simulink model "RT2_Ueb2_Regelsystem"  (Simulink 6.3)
settings: Solver=ode45  StartTime=0.0  StopTime=tfin  RelTol=1e-3
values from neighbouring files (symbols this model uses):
  a = ###    [RT2_Ueb2A1.m]
  b = 1    [RT2_Ueb2A1.m]
  c = 0    [RT2_Ueb2A1.m]
  kp = ###    [RT2_Ueb2A1.m]    (also in RT2_Ueb2A2.m)
  Td = ###    [RT2_Ueb2A1.m]    (also in RT2_Ueb2A2.m = 1/2*(tan(psi-phip)*(rps/rp-phips*tan(phi-phip))+     tan(phi)
  Ti = ###    [RT2_Ueb2A1.m]    (also in RT2_Ueb2A2.m = 1/(Td*wc^2-tan(phi-phip)*wc))
  u_low = -4    [RT2_Ueb2A1.m]
  u_up = 4    [RT2_Ueb2A1.m]
libraries: cstblocks x3

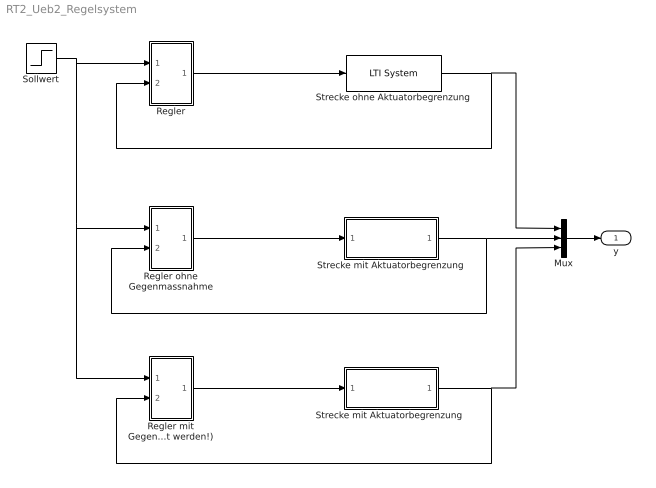
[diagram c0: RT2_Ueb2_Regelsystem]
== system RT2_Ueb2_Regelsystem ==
  Mux : Mux  Inputs=3
  Regler : Subsystem
  Regler mit Gegenmassnahme (Nur dieser Block muss verändert werden!) : Subsystem
  Regler ohne Gegenmassnahme : Subsystem
  Sollwert : Step  Time=0  SampleTime=.1
  Strecke mit Aktuatorbegrenzung : Subsystem
  "Strecke mit Aktuatorbegrenzung " : Subsystem
  Strecke ohne Aktuatorbegrenzung : cstblocks/LTI System  sys=P  IC=[]
  y : Outport
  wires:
  Strecke ohne Aktuatorbegrenzung/1 -> Regler/2(y), Mux/1
  Sollwert/1 -> Regler/1(r), Regler mit Gegenmassnahme (Nur dieser Block muss verändert werden!)/1(r), Regler ohne Gegenmassnahme/1(r)
  Regler/1(u) -> Strecke ohne Aktuatorbegrenzung/1
  "Strecke mit Aktuatorbegrenzung "/1(y) -> Regler mit Gegenmassnahme (Nur dieser Block muss verändert werden!)/2(y), Mux/3
  Regler mit Gegenmassnahme (Nur dieser Block muss verändert werden!)/1(u) -> "Strecke mit Aktuatorbegrenzung "/1(u)
  Strecke mit Aktuatorbegrenzung/1(y) -> Regler ohne Gegenmassnahme/2(y), Mux/2
  Regler ohne Gegenmassnahme/1(u) -> Strecke mit Aktuatorbegrenzung/1(u)
  Mux/1 -> y/1

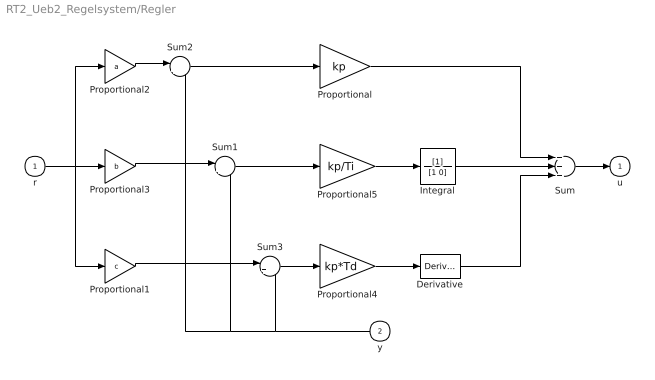
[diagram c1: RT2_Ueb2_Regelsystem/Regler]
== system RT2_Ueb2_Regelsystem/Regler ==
  r : Inport
  y : Inport  Orientation=left  Port=2
  Derivative : Derivative
  Integral : TransferFcn  Denominator=[1 0]
  Proportional : Gain  Gain=kp
  Proportional1 : Gain  Gain=c
  Proportional2 : Gain  Gain=a
  Proportional3 : Gain  Gain=b
  Proportional4 : Gain  Gain=kp*Td
  Proportional5 : Gain  Gain=kp/Ti
  Sum : Sum  Inputs=+++
  Sum1 : Sum  Inputs=|+-
  Sum2 : Sum  Inputs=|+-
  Sum3 : Sum  Inputs=|+-
  u : Outport  InitialOutput=0
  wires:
  Proportional/1 -> Sum/1
  Integral/1 -> Sum/2
  Derivative/1 -> Sum/3
  Sum1/1 -> Proportional5/1
  Sum/1 -> u/1
  Proportional4/1 -> Derivative/1
  r/1 -> Proportional2/1, Proportional1/1, Proportional3/1
  Sum2/1 -> Proportional/1
  Proportional2/1 -> Sum2/1
  Proportional1/1 -> Sum3/1
  Proportional3/1 -> Sum1/1
  Proportional5/1 -> Integral/1
  Sum3/1 -> Proportional4/1
  y/1 -> Sum3/2, Sum1/2, Sum2/2

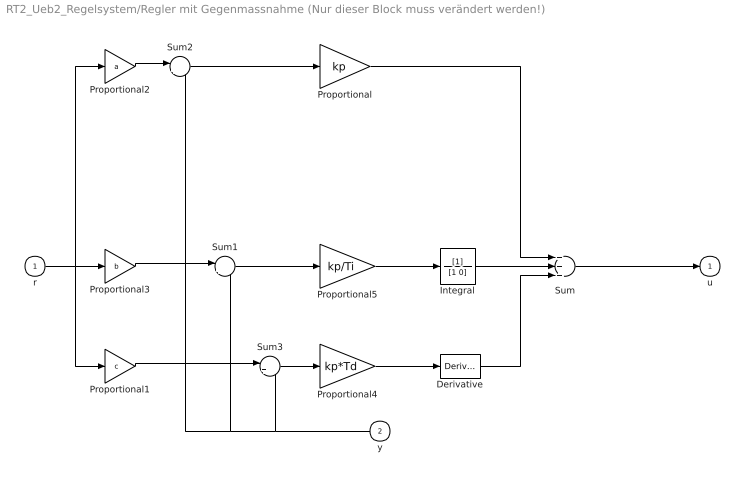
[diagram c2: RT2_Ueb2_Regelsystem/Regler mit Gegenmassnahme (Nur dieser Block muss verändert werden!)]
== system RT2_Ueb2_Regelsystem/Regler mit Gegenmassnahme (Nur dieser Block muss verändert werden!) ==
  r : Inport
  y : Inport  Orientation=left  Port=2
  Derivative : Derivative
  Integral : TransferFcn  Denominator=[1 0]
  Proportional : Gain  Gain=kp
  Proportional1 : Gain  Gain=c
  Proportional2 : Gain  Gain=a
  Proportional3 : Gain  Gain=b
  Proportional4 : Gain  Gain=kp*Td
  Proportional5 : Gain  Gain=kp/Ti
  Sum : Sum  Inputs=+++
  Sum1 : Sum  Inputs=|+-
  Sum2 : Sum  Inputs=|+-
  Sum3 : Sum  Inputs=|+-
  u : Outport  InitialOutput=0
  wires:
  y/1 -> Sum2/2, Sum1/2, Sum3/2
  Sum3/1 -> Proportional4/1
  Proportional5/1 -> Integral/1
  Proportional3/1 -> Sum1/1
  Proportional1/1 -> Sum3/1
  Proportional2/1 -> Sum2/1
  Sum2/1 -> Proportional/1
  r/1 -> Proportional3/1, Proportional1/1, Proportional2/1
  Proportional4/1 -> Derivative/1
  Sum/1 -> u/1
  Sum1/1 -> Proportional5/1
  Derivative/1 -> Sum/3
  Integral/1 -> Sum/2
  Proportional/1 -> Sum/1

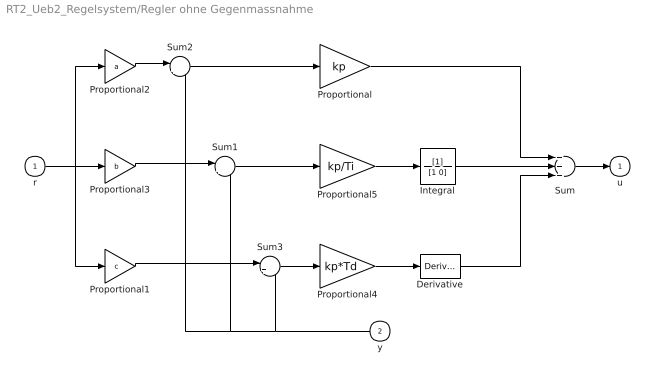
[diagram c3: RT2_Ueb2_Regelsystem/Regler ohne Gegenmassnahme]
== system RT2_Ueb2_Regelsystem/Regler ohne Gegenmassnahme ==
  r : Inport
  y : Inport  Orientation=left  Port=2
  Derivative : Derivative
  Integral : TransferFcn  Denominator=[1 0]
  Proportional : Gain  Gain=kp
  Proportional1 : Gain  Gain=c
  Proportional2 : Gain  Gain=a
  Proportional3 : Gain  Gain=b
  Proportional4 : Gain  Gain=kp*Td
  Proportional5 : Gain  Gain=kp/Ti
  Sum : Sum  Inputs=+++
  Sum1 : Sum  Inputs=|+-
  Sum2 : Sum  Inputs=|+-
  Sum3 : Sum  Inputs=|+-
  u : Outport  InitialOutput=0
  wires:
  y/1 -> Sum2/2, Sum1/2, Sum3/2
  Sum3/1 -> Proportional4/1
  Proportional5/1 -> Integral/1
  Proportional3/1 -> Sum1/1
  Proportional1/1 -> Sum3/1
  Proportional2/1 -> Sum2/1
  Sum2/1 -> Proportional/1
  r/1 -> Proportional3/1, Proportional1/1, Proportional2/1
  Proportional4/1 -> Derivative/1
  Sum/1 -> u/1
  Sum1/1 -> Proportional5/1
  Derivative/1 -> Sum/3
  Integral/1 -> Sum/2
  Proportional/1 -> Sum/1

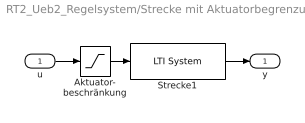
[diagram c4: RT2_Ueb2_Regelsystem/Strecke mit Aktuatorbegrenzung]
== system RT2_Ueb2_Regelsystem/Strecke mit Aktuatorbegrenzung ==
  u : Inport
  Aktuator- beschränkung : Saturate  UpperLimit=u_up  LowerLimit=u_low
  Strecke1 : cstblocks/LTI System  sys=P  IC=[]
  y : Outport
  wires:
  Strecke1/1 -> y/1
  u/1 -> Aktuator- beschränkung/1
  Aktuator- beschränkung/1 -> Strecke1/1

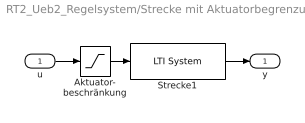
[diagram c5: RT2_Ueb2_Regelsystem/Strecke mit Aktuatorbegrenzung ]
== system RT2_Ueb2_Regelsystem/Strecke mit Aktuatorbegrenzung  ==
  u : Inport
  Aktuator- beschränkung : Saturate  UpperLimit=u_up  LowerLimit=u_low
  Strecke1 : cstblocks/LTI System  sys=P  IC=[]
  y : Outport
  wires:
  Aktuator- beschränkung/1 -> Strecke1/1
  u/1 -> Aktuator- beschränkung/1
  Strecke1/1 -> y/1
